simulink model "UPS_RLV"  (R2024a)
settings: Solver=VariableStepAuto  StartTime=0.0  StopTime=3000  RelTol=1e-3
undefined symbols (not defined in the file): Ion, Lithium
libraries: spsBatteryLib x1, spsControlledCurrentSourceLib x1, spsIdealSwitchLib x1, simulink x1, sps_lib x1

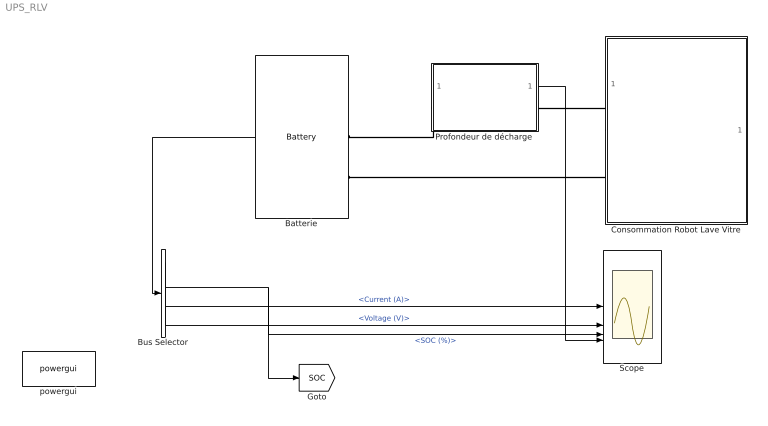
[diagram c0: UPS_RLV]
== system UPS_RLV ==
  Batterie : spsBatteryLib/Battery  BatType=Lithium-Ion  ShowTempParam=off  ThermalPreset=no  ShowAgeParam=off  NomV=12  NomQ=1  SOC=100  Batt_Tr=30  PresetModel=on  MaxQ=1  MinV=9  FullV=13.9678  Dis_rate=0.43478  R=0.12  Normal_OP=0.90435  expZone="[12.9646    0.0491304]"  current=[6.5 13 32.5]  Units=Time  Tci=20  NomT=20  T2=-30  MaxQ2=4.8  FullV2=7.1  Normal_OP2=5.655  expZone2="[6.58           1]"  Rca=0.6  ti=2000  Dp=0  Neq0=0  Tsim=1e6  Ta1=25  Qeol=5.4*0.9  Reol=0.013333*1.2  Char_age=[2.3478, 3]  Dis_age=[2.3478, 10]  N1=1500  N2=10500  N3=1000  N4=1400  Ta2=45  N5=950
  Bus Selector : BusSelector  OutputSignals=Current (A),Voltage (V),SOC (%)
  Consommation Robot Lave Vitre : Subsystem
  Profondeur de décharge : Subsystem
  Scope : Scope  NumInputPorts=4
  powergui : sps_lib/powergui  Priority=1  SimulationMode=Continuous  SampleTime=50e-6  frequency=60  Iterations=50  frequencyindice=0  Pbase=100e6  ErrMax=1e-4  UnitsV=kV  UnitsW=MW  buscounter=0  FunctionMessages=off  echomessages=off  EnableUseOfTLC=off  CurrentSourceSwitches=off  DisableSnubberDevices=off  DisableRonSwitches=off  DisableVfSwitches=off  DisplayEquations=off  AutomaticDiscreteSolvers=off  SolverType=Tustin/Backward Euler (TBE)  Interpol=off  ExternalGateDelay=off  methode=off  Ts=100  x0status=blocks  SPID=on  SwTol=0  HookPort=off  NonlinearTolerance=1e-4  nMaxIteration=100  ContinueOnMaxIteration=off  RestoreLinks=warning  ResistiveCurrentMeasurement=off  Frange=[0:2:500]  Ylog=off  Xlog=on  ShowGrid=off  save=off  variable=ZData  structure=0  ZoomFFT=off  StartTime=0.0  cycles=1  DisplayStyle=1  fundamental=60  FreqAxis=off  MaxFrequency=1000  frequencyindicesteady=1  RmsSteady=1  display=off
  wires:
  Bus Selector/3 -> [SOC], Scope/3  "<SOC (%)>"
  Bus Selector/1 -> Scope/1  "<Current (A)>"
  Batterie/1 -> Bus Selector/1
  Bus Selector/2 -> Scope/2  "<Voltage (V)>"
  Profondeur de décharge/1(Déchargé ?) -> Scope/4
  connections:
  Consommation Robot Lave Vitre/LConn2 -- Batterie/LConn2
  Consommation Robot Lave Vitre/LConn1 -- Profondeur de décharge/RConn1
  Profondeur de décharge/LConn1 -- Batterie/LConn1

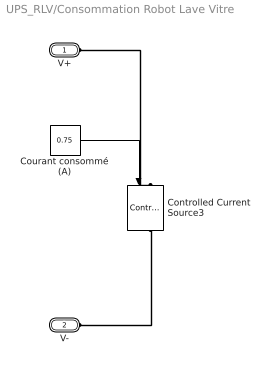
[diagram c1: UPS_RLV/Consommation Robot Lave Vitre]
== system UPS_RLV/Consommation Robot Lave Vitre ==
  Controlled Current Source3 : spsControlledCurrentSourceLib/Controlled Current Source  Initialize=on  Source_Type=DC  Amplitude=0  Phase=0  Frequency=0  Measurements=None
  Courant consommé (A) : Constant  Value=0.75
  V+ : PMIOPort  Side=Left
  V- : PMIOPort  Port=2  Side=Left
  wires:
  Courant consommé (A)/1 -> Controlled Current Source3/1
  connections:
  Controlled Current Source3/RConn1 -- V-/RConn1
  V+/RConn1 -- Controlled Current Source3/LConn1

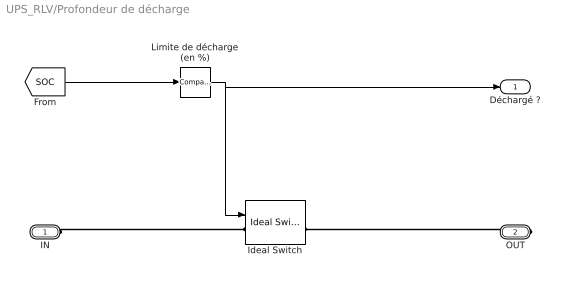
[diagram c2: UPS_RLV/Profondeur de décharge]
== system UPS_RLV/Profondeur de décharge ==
  Ideal Switch : spsIdealSwitchLib/Ideal Switch  Ron=0.001  Lon=0  IC=1  Rs=1e5  Cs=inf  Measurements=on
  Limite de décharge (en %) : simulink/Logic and Bit Operations/Compare To Constant  relop=>=  const=20  OutDataTypeStr=uint8
  IN : PMIOPort  Side=Left
  OUT : PMIOPort  Port=2  Side=Right
  Déchargé ? : Outport
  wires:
  Limite de décharge (en %)/1 -> Déchargé ?/1, Ideal Switch/1
  [SOC] -> Limite de décharge (en %)/1
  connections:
  IN/RConn1 -- Ideal Switch/LConn1
  OUT/RConn1 -- Ideal Switch/RConn1
